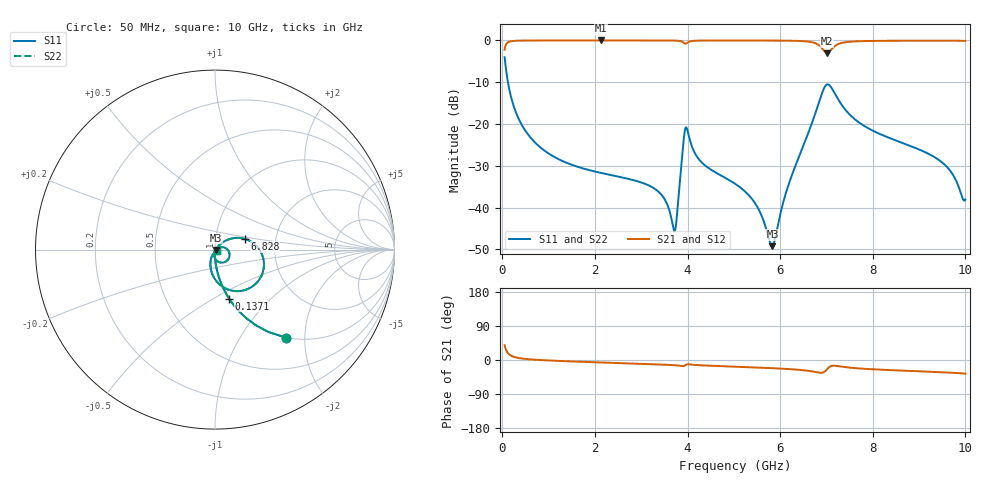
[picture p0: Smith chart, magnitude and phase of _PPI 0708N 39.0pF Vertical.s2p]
! S-Parameter data specifications (vertical orientation):
! Substrate: 40-mil Rogers 3003C, Substrate thickness, H=1.016mm, Dielectric constant, Er=3, Conductor thickness, T_mtl=0.043mm, Loss Tangent, Tand=0.003
! PCB Mounting Pad Footprint: Pad width, PadW=2.54mm , Pad length, PadL=0.51mm , Pad gap, PadG (edge-to-edge)=0.71mm , Reference planes=1.73mm apart
! Created Fri Jan 19 09:05:43 2018
# GHz S MA R 50
! 2 Port Network Data from SP1.SP block
! freq  magS11  angS11  magS21  angS21  magS12  angS12  magS22  angS22
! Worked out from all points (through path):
!   801 points, 50 MHz to 10 GHz, reference 50 ohm
!   highest |S21| = -0.01 dB at 2.139 GHz (marker M1); lowest = -3.1 dB at 7.015 GHz (marker M2)
!   group delay of S21, straight-line fit = 10.5 ps
!   lowest |S11| = -49.2 dB at 5.833 GHz (marker M3), VSWR 1.01, Z = 50.3 - j0.153 ohm
!   |S11| at or under -10 dB: 122.1 MHz to end of sweep
!   |S22| runs from -49.2 to -4.0 dB; largest |S21 - S12| = 0
!   S11 on the Smith chart (normalised r, x): 50 MHz: 1.00, -1.62; 137.1 MHz: 1.00, -0.59; 6.828 GHz: 1.38, +0.17; 10 GHz: 1.02, -0.02
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0.05  0.6305 -51.1  0.776 38.9  0.776 38.9  0.6305 -51.1
0.1370625  0.2845 -74.0  0.9585 16.0  0.9585 16.0  0.2845 -74.0
0.323625  0.1257 -83.9  0.9919 6.0  0.9919 6.0  0.1257 -83.9
0.6345625  0.06634 -88.4  0.9975 1.4  0.9975 1.4  0.06634 -88.4
1.716625  0.02973 -94.0  0.9991 -4.8  0.9991 -4.8  0.02973 -94.0
2.1395  0.02594 -95.6  0.9991 -6.6  0.9991 -6.6  0.02594 -95.6
3.370812  0.01554 -97.6  0.9986 -11.7  0.9986 -11.7  0.01554 -97.6
3.719063  0.005187 -38.3  0.9951 -13.8  0.9951 -13.8  0.005187 -38.3
3.918063  0.06542 3.9  0.938 -15.9  0.938 -15.9  0.06542 3.9
3.98025  0.08998 -47.8  0.9256 -11.8  0.9256 -11.8  0.08998 -47.8
4.27875  0.03601 -97.6  0.9952 -13.9  0.9952 -13.9  0.03601 -97.6
5.025  0.01929 -102.5  0.9979 -17.6  0.9979 -17.6  0.01929 -102.5
5.47275  0.01096 -98.1  0.9975 -19.7  0.9975 -19.7  0.01096 -98.1
5.833437  0.003457 -26.1  0.9963 -21.6  0.9963 -21.6  0.003457 -26.1
6.16925  0.01792 44.6  0.993 -23.7  0.993 -23.7  0.01792 44.6
6.691625  0.1045 35.0  0.9512 -30.1  0.9512 -30.1  0.1045 35.0
6.828437  0.1756 19.9  0.8844 -33.2  0.8844 -33.2  0.1756 19.9
7.015  0.2974 -30.0  0.7034 -24.0  0.7034 -24.0  0.2974 -30.0
7.338375  0.1666 -89.6  0.9351 -17.8  0.9351 -17.8  0.1666 -89.6
8.345812  0.06853 -111.0  0.9908 -26.5  0.9908 -26.5  0.06853 -111.0
9.490063  0.03498 -114.4  0.9942 -32.3  0.9942 -32.3  0.03498 -114.4
10  0.01253 -42.3  0.9871 -35.9  0.9871 -35.9  0.01253 -42.3
